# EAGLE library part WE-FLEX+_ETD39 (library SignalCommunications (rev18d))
WE-FLEX+ Flexible Transformer for DC/DC Converter Characteristics Transformer with 6 identical windings Power up to 300 W possible Isolation voltage 500 VDC Low leakage inductance Operating temperature: –40 °C to +125 °C Applications All kind of switching regulators -Flyback converters -Forward converters -Push-pull converters -Step-up/step-down converters -SEPIC converter Details see: http://katalog.we-online.de/en/pbs/WE-FLEX-PLUS Updated by Dan Xu 2014-07-07 2014 (C) Wurth Elektronik
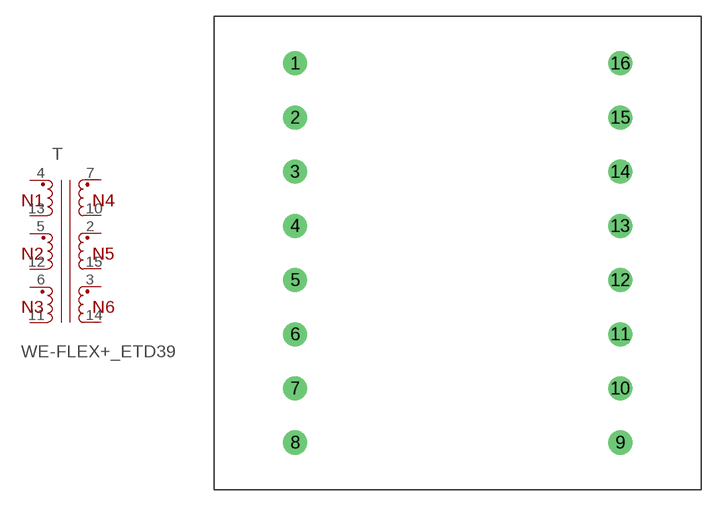
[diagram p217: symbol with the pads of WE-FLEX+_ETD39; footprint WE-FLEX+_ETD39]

Designator prefix T

## WE-FLEX+_ETD39_749197301, WE-FLEX+_ETD39_749197311, WE-FLEX+_ETD39_749197321, WE-FLEX+_ETD39_749197331, WE-FLEX+_ETD39_749197341  [WE-FLEX+_ETD39]
2  4  pas
3  6  pas
4  1  pas
5  11  pas
6  9  pas
7  2  pas
10  3  pas
11  8  pas
12  10  pas
13  12  pas
14  7  pas
15  5  pas

## Footprint WE-FLEX+_ETD39 (pad centres in mm)
Transformer, ETD39 THT 16Pin
drill 1.5: 1 -15.24,17.78; 2 -15.24,12.7; 3 -15.24,7.62; 4 -15.24,2.54; 5 -15.24,-2.54; 6 -15.24,-7.62; 7 -15.24,-12.7; 8 -15.24,-17.78; 9 15.24,-17.78; 10 15.24,-12.7; 11 15.24,-7.62; 12 15.24,-2.54; 13 15.24,2.54; 14 15.24,7.62; 15 15.24,12.7; 16 15.24,17.78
